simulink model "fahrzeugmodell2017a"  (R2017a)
settings: Solver=FixedStepDiscrete  StartTime=0.0  StopTime=40  FixedStep=T  RelTol=1e-3  EnableMultiTasking=on
undefined symbols (not defined in the file): DiscIntNeverNeededParam, PAR_Darstellung_Schalter_EIN_bit, PAR_FZG_abstand_sensor_VA_f64, PAR_FZG_psi0_I_f64, PAR_FZG_radstand_f64, PAR_FZG_spurweite_f64, PAR_FZG_x0_I_f64, PAR_FZG_xD0_I_f64, PAR_FZG_y0_I_f64, PAR_FZG_yD0_I_f64, PAR_VIS_Anzahl_Schritte_n

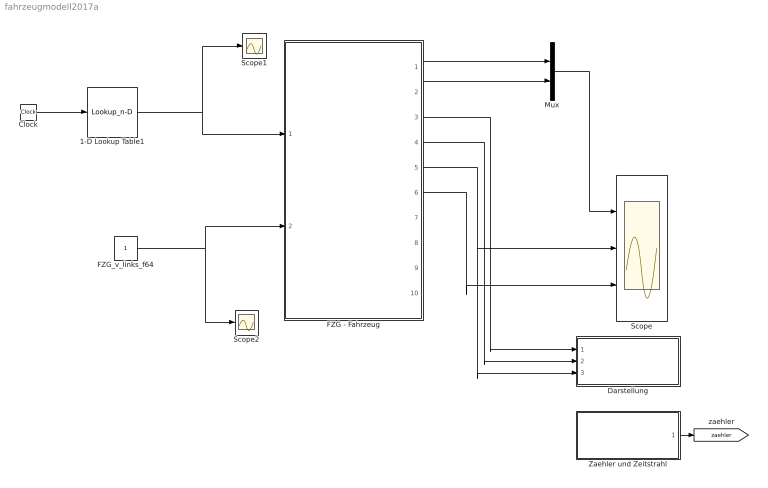
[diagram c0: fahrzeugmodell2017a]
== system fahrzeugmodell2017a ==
  1-D Lookup Table1 : Lookup_n-D  NumberOfTableDimensions=1  BreakpointsForDimension1=[0 20 20.1 40]  Table=[1.2 1.2 0.8 0.8]  InternalRulePriority=Speed  RndMeth=Simplest
  Clock : Clock
  Darstellung : Subsystem
  FZG - Fahrzeug : Subsystem
  FZG_v_links_f64 : Constant
  Mux : Mux  Inputs=2
  Scope : Scope  NumInputPorts=3
  Scope1 : Scope
  Scope2 : Scope
  Zaehler und Zeitstrahl : Subsystem
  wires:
  FZG - Fahrzeug/1(FZG_vx_I_f64) -> Mux/1
  FZG - Fahrzeug/2(FZG_vy_I_f64) -> Mux/2
  FZG - Fahrzeug/4(FZG_y_I_f64) -> Darstellung/2(y)
  FZG - Fahrzeug/5(FZG_psi_f64) -> Darstellung/3(psi), Scope/2
  FZG - Fahrzeug/6(FZG_psip_f64) -> Scope/3
  Mux/1 -> Scope/1
  Zaehler und Zeitstrahl/1(zaehler) -> [zaehler]
  FZG - Fahrzeug/3(FZG_x_I_f64) -> Darstellung/1(x)
  Clock/1 -> 1-D Lookup Table1/1
  FZG_v_links_f64/1 -> Scope2/1, FZG - Fahrzeug/2(FZG_v_links_f64)
  1-D Lookup Table1/1 -> Scope1/1, FZG - Fahrzeug/1(FZG_v_rechts_f64)

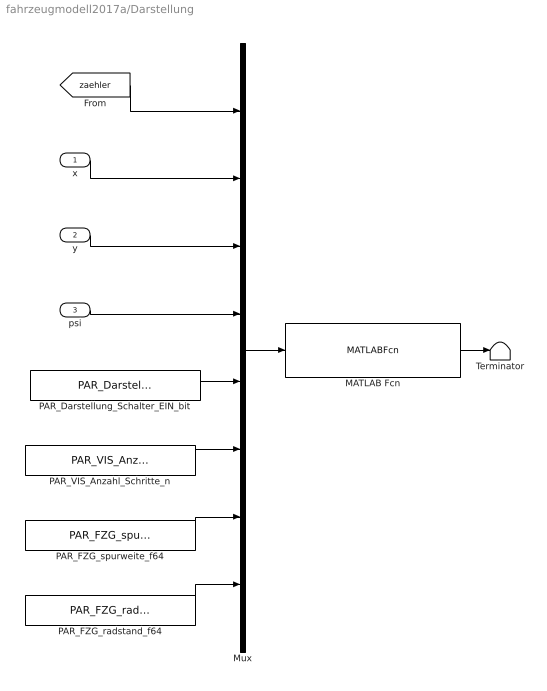
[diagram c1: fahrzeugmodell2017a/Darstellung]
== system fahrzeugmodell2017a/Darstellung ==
  x : Inport
  y : Inport  Port=2
  psi : Inport  Port=3
  MATLAB Fcn : MATLABFcn  InitFcn=temp_zaehler = [];  MATLABFcn=funktion_simulink_simultan_draufsicht
  Mux : Mux  Inputs=8
  PAR_Darstellung_Schalter_EIN_bit : Constant  Value=PAR_Darstellung_Schalter_EIN_bit
  PAR_FZG_radstand_f64 : Constant  Value=PAR_FZG_radstand_f64
  PAR_FZG_spurweite_f64 : Constant  Value=PAR_FZG_spurweite_f64
  PAR_VIS_Anzahl_Schritte_n : Constant  Value=PAR_VIS_Anzahl_Schritte_n
  Terminator : Terminator
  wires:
  MATLAB Fcn/1 -> Terminator/1
  Mux/1 -> MATLAB Fcn/1
  [zaehler] -> Mux/1
  PAR_Darstellung_Schalter_EIN_bit/1 -> Mux/5
  psi/1 -> Mux/4
  y/1 -> Mux/3
  x/1 -> Mux/2
  PAR_VIS_Anzahl_Schritte_n/1 -> Mux/6
  PAR_FZG_spurweite_f64/1 -> Mux/7
  PAR_FZG_radstand_f64/1 -> Mux/8

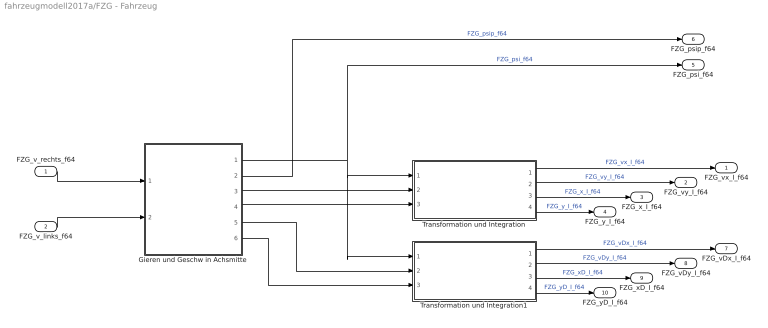
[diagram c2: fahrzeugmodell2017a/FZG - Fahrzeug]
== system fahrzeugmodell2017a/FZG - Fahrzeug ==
  FZG_v_rechts_f64 : Inport
  FZG_v_links_f64 : Inport  Port=2
  Gieren und Geschw in Achsmitte : Subsystem
  Transformation und Integration : Subsystem
  Transformation und Integration1 : Subsystem
  FZG_vx_I_f64 : Outport
  FZG_vy_I_f64 : Outport  Port=2
  FZG_x_I_f64 : Outport  Port=3
  FZG_y_I_f64 : Outport  Port=4
  FZG_psi_f64 : Outport  Port=5
  FZG_psip_f64 : Outport  Port=6
  FZG_vDx_I_f64 : Outport  Port=7
  FZG_vDy_I_f64 : Outport  Port=8
  FZG_xD_I_f64 : Outport  Port=9
  FZG_yD_I_f64 : Outport  Port=10
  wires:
  FZG_v_rechts_f64/1 -> Gieren und Geschw in Achsmitte/1(FZG_v_rechts_f64)
  Gieren und Geschw in Achsmitte/1(psi) -> Transformation und Integration1/1(psi), Transformation und Integration/1(psi), FZG_psi_f64/1  "FZG_psi_f64"
  FZG_v_links_f64/1 -> Gieren und Geschw in Achsmitte/2(FZG_v_links_f64)
  Gieren und Geschw in Achsmitte/2(psip) -> FZG_psip_f64/1  "FZG_psip_f64"
  Transformation und Integration/1(FZG_vx_I_f64) -> FZG_vx_I_f64/1  "FZG_vx_I_f64"
  Transformation und Integration/2(FZG_vy_I_f64) -> FZG_vy_I_f64/1  "FZG_vy_I_f64"
  Gieren und Geschw in Achsmitte/3(v_mitte_x_K) -> Transformation und Integration/2(v_mitte_x_K)
  Transformation und Integration/3(FZG_x_I_f64) -> FZG_x_I_f64/1  "FZG_x_I_f64"
  Transformation und Integration/4(FZG_y_I_f64) -> FZG_y_I_f64/1  "FZG_y_I_f64"
  Gieren und Geschw in Achsmitte/4("v_mitte_y_K ") -> Transformation und Integration/3(v_mitte_y_K)
  Transformation und Integration1/4(FZG_y_I_f64) -> FZG_yD_I_f64/1  "FZG_yD_I_f64"
  Transformation und Integration1/3(FZG_x_I_f64) -> FZG_xD_I_f64/1  "FZG_xD_I_f64"
  Transformation und Integration1/2(FZG_vy_I_f64) -> FZG_vDy_I_f64/1  "FZG_vDy_I_f64"
  Transformation und Integration1/1(FZG_vx_I_f64) -> FZG_vDx_I_f64/1  "FZG_vDx_I_f64"
  Gieren und Geschw in Achsmitte/5(v_D_x_K) -> Transformation und Integration1/2(v_D_x_K)
  Gieren und Geschw in Achsmitte/6(v_D_y_K) -> Transformation und Integration1/3(v_D_y_K)

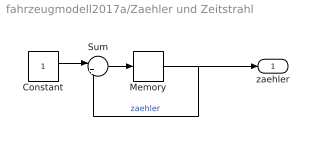
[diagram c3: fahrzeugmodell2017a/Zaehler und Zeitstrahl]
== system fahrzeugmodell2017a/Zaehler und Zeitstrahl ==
  Constant : Constant
  Memory : Memory  X0=1
  Sum : Sum  Inputs=|++
  zaehler : Outport
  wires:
  Sum/1 -> Memory/1
  Memory/1 -> Sum/2, zaehler/1  "zaehler"
  Constant/1 -> Sum/1

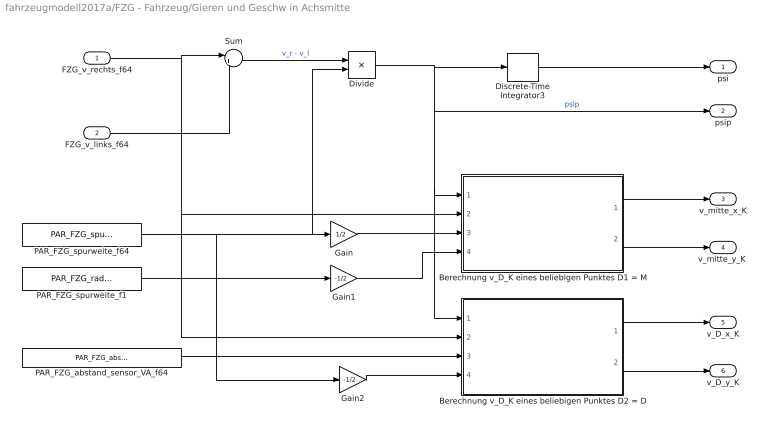
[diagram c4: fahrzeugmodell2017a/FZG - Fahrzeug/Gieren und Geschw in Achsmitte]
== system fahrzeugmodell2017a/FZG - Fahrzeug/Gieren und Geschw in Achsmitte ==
  FZG_v_rechts_f64 : Inport
  FZG_v_links_f64 : Inport  Port=2
  Berechnung v_D_K eines beliebigen Punktes D1 = M : Subsystem
  Berechnung v_D_K eines beliebigen Punktes D2 = D : Subsystem
  Discrete-Time Integrator3 : DiscreteIntegrator  InitialCondition=PAR_FZG_psi0_I_f64  SampleTime=-1  ICPrevOutput=DiscIntNeverNeededParam  ICPrevScaledInput=DiscIntNeverNeededParam
  Divide : Product  Inputs=*/
  Gain : Gain  Gain=1/2
  Gain1 : Gain  Gain=-1/2
  Gain2 : Gain  Gain=-1/2
  PAR_FZG_abstand_sensor_VA_f64 : Constant  Value=PAR_FZG_abstand_sensor_VA_f64
  PAR_FZG_spurweite_f1 : Constant  Value=PAR_FZG_radstand_f64
  PAR_FZG_spurweite_f64 : Constant  Value=PAR_FZG_spurweite_f64
  Sum : Sum  Inputs=|+-
  psi : Outport
  psip : Outport  Port=2
  v_mitte_x_K : Outport  Port=3
  "v_mitte_y_K " : Outport  Port=4
  v_D_x_K : Outport  Port=5
  v_D_y_K : Outport  Port=6
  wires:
  Sum/1 -> Divide/1  "v_r - v_l"
  FZG_v_links_f64/1 -> Sum/2
  PAR_FZG_spurweite_f64/1 -> Gain2/1, Gain/1, Divide/2
  Discrete-Time Integrator3/1 -> psi/1
  FZG_v_rechts_f64/1 -> Berechnung v_D_K eines beliebigen Punktes D2 = D/2(v_rechts_x_K), Berechnung v_D_K eines beliebigen Punktes D1 = M/2(v_rechts_x_K), Sum/1
  Divide/1 -> Berechnung v_D_K eines beliebigen Punktes D2 = D/1(psip), Berechnung v_D_K eines beliebigen Punktes D1 = M/1(psip), psip/1, Discrete-Time Integrator3/1  "psip"
  PAR_FZG_spurweite_f1/1 -> Gain1/1
  Berechnung v_D_K eines beliebigen Punktes D1 = M/1(v_D_x_K) -> v_mitte_x_K/1
  Berechnung v_D_K eines beliebigen Punktes D1 = M/2(v_D_y_K) -> "v_mitte_y_K "/1
  Gain/1 -> Berechnung v_D_K eines beliebigen Punktes D1 = M/3(r_RD_x_K)
  Gain1/1 -> Berechnung v_D_K eines beliebigen Punktes D1 = M/4(r_RD_y_K)
  Berechnung v_D_K eines beliebigen Punktes D2 = D/1(v_D_x_K) -> v_D_x_K/1
  Berechnung v_D_K eines beliebigen Punktes D2 = D/2(v_D_y_K) -> v_D_y_K/1
  PAR_FZG_abstand_sensor_VA_f64/1 -> Berechnung v_D_K eines beliebigen Punktes D2 = D/3(r_RD_x_K)
  Gain2/1 -> Berechnung v_D_K eines beliebigen Punktes D2 = D/4(r_RD_y_K)

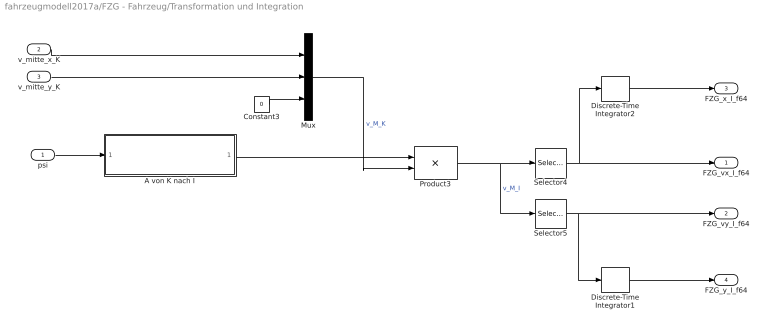
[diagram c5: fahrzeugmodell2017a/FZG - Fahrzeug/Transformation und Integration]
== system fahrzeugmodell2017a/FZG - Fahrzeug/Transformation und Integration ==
  psi : Inport
  v_mitte_x_K : Inport  Port=2
  v_mitte_y_K : Inport  Port=3
  A von K nach I : Subsystem
  Constant3 : Constant  Value=0
  Discrete-Time Integrator1 : DiscreteIntegrator  InitialCondition=PAR_FZG_y0_I_f64  SampleTime=-1  ICPrevOutput=DiscIntNeverNeededParam  ICPrevScaledInput=DiscIntNeverNeededParam
  Discrete-Time Integrator2 : DiscreteIntegrator  InitialCondition=PAR_FZG_x0_I_f64  SampleTime=-1  ICPrevOutput=DiscIntNeverNeededParam  ICPrevScaledInput=DiscIntNeverNeededParam
  Mux : Mux  Inputs=3
  Product3 : Product  Multiplication=Matrix(*)
  Selector4 : Selector  InputPortWidth=3  IndexOptions=Index vector (dialog)  Indices=[1]  OutputSizes=1
  Selector5 : Selector  InputPortWidth=3  IndexOptions=Index vector (dialog)  Indices=[2]  OutputSizes=1
  FZG_vx_I_f64 : Outport
  FZG_vy_I_f64 : Outport  Port=2
  FZG_x_I_f64 : Outport  Port=3
  FZG_y_I_f64 : Outport  Port=4
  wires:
  Constant3/1 -> Mux/3
  v_mitte_y_K/1 -> Mux/2
  Mux/1 -> Product3/2  "v_M_K"
  A von K nach I/1(A_von_2_nach_1) -> Product3/1
  Product3/1 -> Selector4/1, Selector5/1  "v_M_I"
  Selector5/1 -> Discrete-Time Integrator1/1, FZG_vy_I_f64/1
  v_mitte_x_K/1 -> Mux/1
  psi/1 -> A von K nach I/1(psi)
  Selector4/1 -> Discrete-Time Integrator2/1, FZG_vx_I_f64/1
  Discrete-Time Integrator2/1 -> FZG_x_I_f64/1
  Discrete-Time Integrator1/1 -> FZG_y_I_f64/1

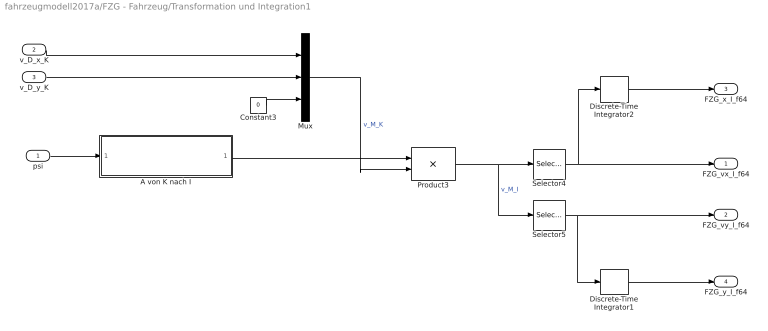
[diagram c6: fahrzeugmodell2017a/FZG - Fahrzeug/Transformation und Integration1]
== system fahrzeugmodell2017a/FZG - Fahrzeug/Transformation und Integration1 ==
  psi : Inport
  v_D_x_K : Inport  Port=2
  v_D_y_K : Inport  Port=3
  A von K nach I : Subsystem
  Constant3 : Constant  Value=0
  Discrete-Time Integrator1 : DiscreteIntegrator  InitialCondition=PAR_FZG_yD0_I_f64  SampleTime=-1  ICPrevOutput=DiscIntNeverNeededParam  ICPrevScaledInput=DiscIntNeverNeededParam
  Discrete-Time Integrator2 : DiscreteIntegrator  InitialCondition=PAR_FZG_xD0_I_f64  SampleTime=-1  ICPrevOutput=DiscIntNeverNeededParam  ICPrevScaledInput=DiscIntNeverNeededParam
  Mux : Mux  Inputs=3
  Product3 : Product  Multiplication=Matrix(*)
  Selector4 : Selector  InputPortWidth=3  IndexOptions=Index vector (dialog)  Indices=[1]  OutputSizes=1
  Selector5 : Selector  InputPortWidth=3  IndexOptions=Index vector (dialog)  Indices=[2]  OutputSizes=1
  FZG_vx_I_f64 : Outport
  FZG_vy_I_f64 : Outport  Port=2
  FZG_x_I_f64 : Outport  Port=3
  FZG_y_I_f64 : Outport  Port=4
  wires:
  Discrete-Time Integrator1/1 -> FZG_y_I_f64/1
  Discrete-Time Integrator2/1 -> FZG_x_I_f64/1
  Selector4/1 -> FZG_vx_I_f64/1, Discrete-Time Integrator2/1
  psi/1 -> A von K nach I/1(psi)
  v_D_x_K/1 -> Mux/1
  Selector5/1 -> FZG_vy_I_f64/1, Discrete-Time Integrator1/1
  Product3/1 -> Selector5/1, Selector4/1  "v_M_I"
  A von K nach I/1(A_von_2_nach_1) -> Product3/1
  Mux/1 -> Product3/2  "v_M_K"
  v_D_y_K/1 -> Mux/2
  Constant3/1 -> Mux/3

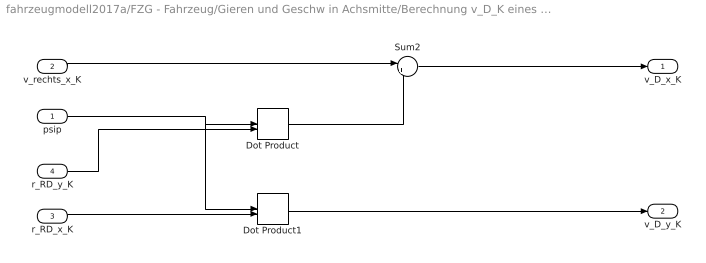
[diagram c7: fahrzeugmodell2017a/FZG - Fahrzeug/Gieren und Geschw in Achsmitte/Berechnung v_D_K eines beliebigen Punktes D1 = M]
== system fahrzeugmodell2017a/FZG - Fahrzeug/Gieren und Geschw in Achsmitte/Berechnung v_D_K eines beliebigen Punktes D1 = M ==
  psip : Inport
  v_rechts_x_K : Inport  Port=2
  r_RD_x_K : Inport  Port=3
  r_RD_y_K : Inport  Port=4
  Dot Product : DotProduct
  Dot Product1 : DotProduct
  Sum2 : Sum  Inputs=|+-
  v_D_x_K : Outport
  v_D_y_K : Outport  Port=2
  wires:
  r_RD_x_K/1 -> Dot Product1/2
  v_rechts_x_K/1 -> Sum2/1
  psip/1 -> Dot Product1/1, Dot Product/1
  r_RD_y_K/1 -> Dot Product/2
  Dot Product/1 -> Sum2/2
  Dot Product1/1 -> v_D_y_K/1
  Sum2/1 -> v_D_x_K/1

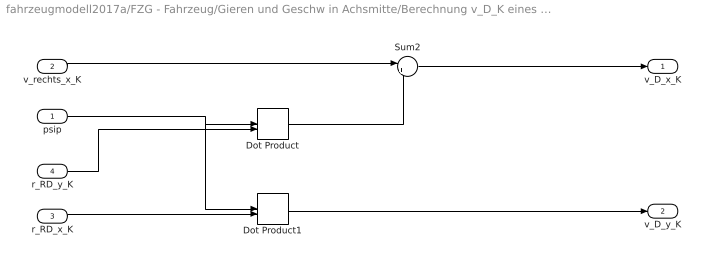
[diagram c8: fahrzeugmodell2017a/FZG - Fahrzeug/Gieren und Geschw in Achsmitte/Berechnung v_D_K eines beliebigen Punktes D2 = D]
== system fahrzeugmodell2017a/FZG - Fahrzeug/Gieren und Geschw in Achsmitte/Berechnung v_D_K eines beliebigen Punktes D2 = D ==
  psip : Inport
  v_rechts_x_K : Inport  Port=2
  r_RD_x_K : Inport  Port=3
  r_RD_y_K : Inport  Port=4
  Dot Product : DotProduct
  Dot Product1 : DotProduct
  Sum2 : Sum  Inputs=|+-
  v_D_x_K : Outport
  v_D_y_K : Outport  Port=2
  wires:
  Sum2/1 -> v_D_x_K/1
  Dot Product1/1 -> v_D_y_K/1
  Dot Product/1 -> Sum2/2
  r_RD_y_K/1 -> Dot Product/2
  psip/1 -> Dot Product/1, Dot Product1/1
  v_rechts_x_K/1 -> Sum2/1
  r_RD_x_K/1 -> Dot Product1/2

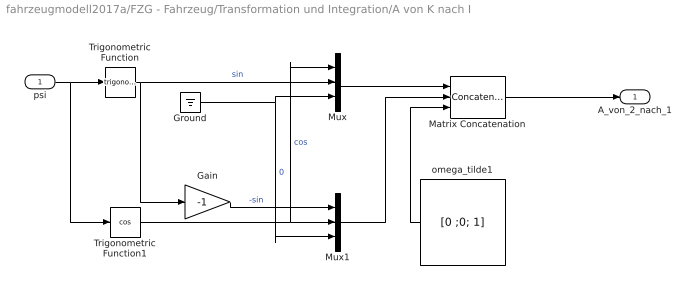
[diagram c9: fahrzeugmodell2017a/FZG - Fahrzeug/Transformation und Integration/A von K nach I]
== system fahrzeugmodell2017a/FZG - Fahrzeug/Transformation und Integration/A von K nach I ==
  psi : Inport
  Gain : Gain  Gain=-1
  Ground : Ground
  Matrix Concatenation : Concatenate  NumInputs=3  Mode=Multidimensional array  ConcatenateDimension=2
  Mux : Mux  Inputs=3
  Mux1 : Mux  Inputs=3
  Trigonometric Function : Trigonometry
  Trigonometric Function1 : Trigonometry  Operator=cos
  omega_tilde1 : Constant  Value=[0 ;0; 1]  VectorParams1D=off
  A_von_2_nach_1 : Outport
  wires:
  Trigonometric Function/1 -> Gain/1, Mux/2  "sin"
  Gain/1 -> Mux1/1  "-sin"
  Ground/1 -> Mux/3, Mux1/3  "0"
  Mux/1 -> Matrix Concatenation/1
  Mux1/1 -> Matrix Concatenation/2
  omega_tilde1/1 -> Matrix Concatenation/3
  Trigonometric Function1/1 -> Mux1/2, Mux/1  "cos"
  psi/1 -> Trigonometric Function/1, Trigonometric Function1/1
  Matrix Concatenation/1 -> A_von_2_nach_1/1

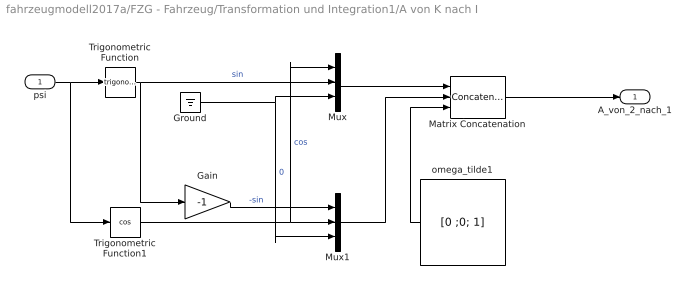
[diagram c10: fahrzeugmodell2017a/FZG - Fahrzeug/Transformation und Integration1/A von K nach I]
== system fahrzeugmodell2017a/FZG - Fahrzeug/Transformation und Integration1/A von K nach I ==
  psi : Inport
  Gain : Gain  Gain=-1
  Ground : Ground
  Matrix Concatenation : Concatenate  NumInputs=3  Mode=Multidimensional array  ConcatenateDimension=2
  Mux : Mux  Inputs=3
  Mux1 : Mux  Inputs=3
  Trigonometric Function : Trigonometry
  Trigonometric Function1 : Trigonometry  Operator=cos
  omega_tilde1 : Constant  Value=[0 ;0; 1]  VectorParams1D=off
  A_von_2_nach_1 : Outport
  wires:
  Matrix Concatenation/1 -> A_von_2_nach_1/1
  psi/1 -> Trigonometric Function1/1, Trigonometric Function/1
  Trigonometric Function1/1 -> Mux/1, Mux1/2  "cos"
  omega_tilde1/1 -> Matrix Concatenation/3
  Mux1/1 -> Matrix Concatenation/2
  Mux/1 -> Matrix Concatenation/1
  Ground/1 -> Mux1/3, Mux/3  "0"
  Gain/1 -> Mux1/1  "-sin"
  Trigonometric Function/1 -> Mux/2, Gain/1  "sin"
